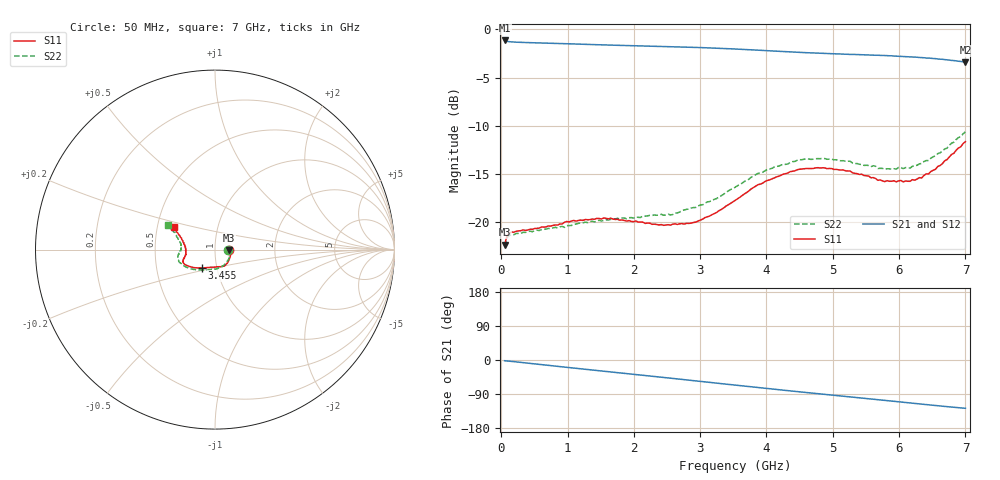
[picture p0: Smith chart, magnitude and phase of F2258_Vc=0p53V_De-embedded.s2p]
! Integrated Device Technology
! Corporate Headquarters
! 6024 Silver Creek Valley Road
! San Jose, CA 95138  USA
! Phone:  1-408-284-8200
! Toll Free:  1-800-223-1366
! Webpage:  http://www.idt.com/
! Timing and RF Division
! 515 Groton Road, Suite 102
! Westford, MA 01886-6024
! Device:  F2258
! Description: Voltage Variable RF Attenuator
! Frequency:  50.0 -  6000.00 MHz
! Package:  3x3 mm Thin QFN Plastic Package: 16 pin
! Ports:  2 RF, 2 DC
!  Pin  1  = NC
!  Pin  2  = NC
!  Pin  3  = RF2  = Port 2
!  Pin  4  = GND
!  Pin  5  = Vdd
!  Pin  6  = NC
!  Pin  7  = VCTRL
!  Pin  8  = NC
!  Pin  9  = GND
!  Pin 10  = RF1  = Port 1
!  Pin 11  = NC
!  Pin 12  = NC
!  Pin 13  = NC
!  Pin 14  = NC
!  Pin 15  = NC
!  Pin 16  = NC
! Vcntrl:  0.530 Volts
! Vdd:  +3.300 Volts
! Current:  1.105 mA
! Data:  The device was measured on a the F2258 evaluation board which has
!  individual transmission lines to the RF pins.  Data was collected
!  using a calibrated network analyzer.  The evaluation board was
!  de-embedded using a TRL calibration technique.
!  The reference plane is the edge of the package pin.
! Misc:  SN 10
!  Action Tracker AT0285
! Date Measured:  2014-12-10
! Date:  2016-01-13  MJV
! Note:
!  Integrated Device Technology supplies this data as a sample of measured
!  data at the package pin for this product.  Your particular data for this
!  product may vary.
!  Data was taken at 25 degrees C.
!  Integrated Device Technology reserves the right to change this data at anytime.
!Freq_(GHz)  S11M_(dB)  S11P_(deg)  S21M_(dB)  S21P_(deg)  S12M_(dB)  S12P_(deg)  S22M_(dB)  S22P_(deg)
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# GHz S dB R 50
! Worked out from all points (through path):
!   201 points, 50 MHz to 7 GHz, reference 50 ohm
!   highest |S21| = -1.14 dB at 50 MHz (marker M1); lowest = -3.4 dB at 7 GHz (marker M2)
!   group delay of S21, straight-line fit = 50.5 ps
!   lowest |S11| = -22.4 dB at 50 MHz (marker M3), VSWR 1.16, Z = 58.2 - j0.458 ohm
!   |S11| at or under -10 dB: start of sweep to end of sweep
!   |S22| runs from -22.5 to -10.6 dB; largest |S21 - S12| = 0.00039
!   S11 on the Smith chart (normalised r, x): 50 MHz: 1.16, -0.01; 3.455 GHz: 0.85, -0.17; 7 GHz: 0.61, +0.16
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0.05  -22.36 -2.9  -1.14 -2.0  -1.14 -2.0  -22.51 -3.0
0.08475  -21.47 -4.8  -1.23 -2.5  -1.23 -2.5  -21.64 -4.9
0.15425  -21.04 -7.5  -1.29 -3.7  -1.29 -3.7  -21.30 -8.4
0.71025  -20.41 -30.9  -1.43 -14.1  -1.43 -14.1  -20.67 -34.6
1.2315  -19.83 -50.7  -1.54 -23.9  -1.54 -23.8  -20.10 -58.1
1.6485  -19.61 -61.4  -1.63 -31.5  -1.62 -31.5  -19.72 -71.2
2.37825  -20.30 -80.4  -1.76 -44.8  -1.76 -44.8  -19.28 -89.8
2.552  -20.32 -86.1  -1.79 -48.0  -1.79 -48.0  -19.27 -95.1
2.93425  -20.01 -102.5  -1.87 -55.1  -1.87 -55.1  -18.49 -108.8
3.247  -19.01 -116.2  -1.94 -61.0  -1.94 -61.0  -17.57 -121.2
3.4555  -18.08 -125.7  -2.01 -64.9  -2.01 -64.9  -16.65 -129.0
3.525  -17.78 -128.1  -2.03 -66.2  -2.03 -66.2  -16.40 -132.1
4.0115  -15.69 -144.0  -2.21 -75.3  -2.21 -75.3  -14.55 -148.2
4.46325  -14.57 -153.4  -2.37 -83.4  -2.37 -83.4  -13.59 -159.7
4.7065  -14.44 -156.7  -2.44 -87.7  -2.44 -87.7  -13.48 -164.1
5.2625  -14.71 -163.3  -2.59 -97.4  -2.59 -97.4  -13.69 -172.5
5.6795  -15.67 -169.4  -2.68 -104.6  -2.68 -104.6  -14.44 -178.2
5.85325  -15.77 -173.6  -2.73 -107.7  -2.73 -107.7  -14.48 177.1
6.166  -15.77 178.3  -2.84 -113.3  -2.84 -113.3  -14.40 171.0
6.33975  -15.42 171.4  -2.92 -116.4  -2.92 -116.4  -13.92 166.5
6.722  -13.52 158.2  -3.15 -123.1  -3.15 -123.0  -12.33 157.2
7  -11.65 151.8  -3.40 -127.4  -3.40 -127.4  -10.64 152.1
